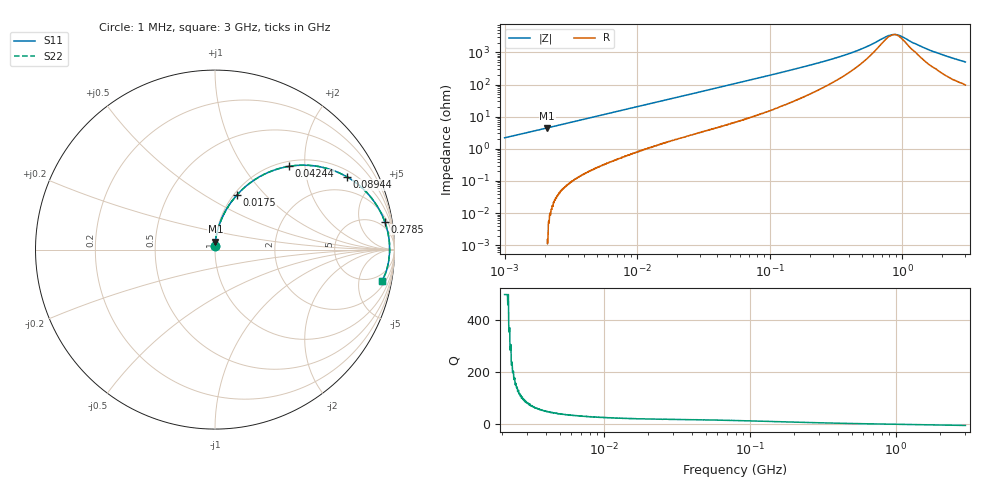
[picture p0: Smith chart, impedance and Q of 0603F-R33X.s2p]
!s-Parameter Generated by FASTRON Sdn. Bhd.
!FASTRON P/N : 0603F-R33X
!Keysight Technologies: E4991B_MY54100416_A.01.15
!Date: Thu Jun 20 13:22:18 2024
!Version  :Rev00  Thu Jun 20 13:22:18 2024
!Data & Calibration Information:
!Freq  S11  S21  S12  S22
!PortZ  Port1:50+j0  Port2:50+j0
!When reading reference impedance value at option line is always used.
! Remarks : This data is being provided solely for informational purposes.
# Hz S dB R 50
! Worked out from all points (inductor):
!   1601 points, 1 MHz to 3 GHz, reference 50 ohm
!   read as one part in series: L = 346 nH near 1.041 MHz
!   highest Q = 372 at 2.097 MHz (marker M1), where L = 340 nH
!   self-resonance near 872.6 MHz
!   S11 on the Smith chart (normalised r, x): 1 MHz: 1.00, +0.04; 17.5 MHz: 1.03, +0.70; 42.44 MHz: 1.10, +1.66; 89.44 MHz: 1.26, +3.46; 278.5 MHz: 3, +11; 3 GHz: 3, -10
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1000000  -33.10 91.5  0.01 -1.3  0.01 -1.3  -33.10 91.5
2097170  -27.00 87.4  -0.01 -2.6  -0.01 -2.6  -27.00 87.4
3804036  -22.00 84.4  -0.04 -4.6  -0.04 -4.6  -22.00 84.4
7550455  -16.30 79.3  -0.15 -8.8  -0.15 -8.8  -16.30 79.3
1.447069e7  -11.10 71.3  -0.46 -16.1  -0.46 -16.1  -11.10 71.3
1.750132e7  -9.70 68.1  -0.64 -19.1  -0.64 -19.1  -9.70 68.1
2.718395e7  -6.66 59.3  -1.30 -27.6  -1.30 -27.6  -6.66 59.3
4.243531e7  -4.12 48.3  -2.53 -38.4  -2.53 -38.4  -4.12 48.3
5.504702e7  -2.98 41.3  -3.59 -45.1  -3.59 -45.1  -2.98 41.3
8.944052e7  -1.52 28.8  -6.31 -56.9  -6.31 -56.9  -1.52 28.8
1.341416e8  -0.85 20.2  -9.21 -64.5  -9.21 -64.5  -0.85 20.2
2.083556e8  -0.49 13.0  -12.90 -69.5  -12.90 -69.5  -0.49 13.0
2.785165e8  -0.37 9.4  -15.60 -70.8  -15.60 -70.8  -0.37 9.4
4.75755e8  -0.26 4.3  -21.90 -66.0  -21.90 -66.0  -0.26 4.3
5.696638e8  -0.25 3.0  -24.70 -59.6  -24.70 -59.6  -0.25 3.0
7.925923e8  -0.24 0.6  -30.70 -21.0  -30.70 -21.0  -0.24 0.6
8.71647e8  -0.24 0.0  -31.40 -0.3  -31.40 -0.3  -0.24 0.0
9.490412e8  -0.24 -0.6  -30.80 20.1  -30.80 20.1  -0.24 -0.6
1.194682e9  -0.26 -2.2  -26.40 51.4  -26.40 51.4  -0.26 -2.2
1.662201e9  -0.28 -4.7  -21.30 65.9  -21.30 65.9  -0.28 -4.7
2.347656e9  -0.36 -7.8  -17.10 69.4  -17.10 69.4  -0.36 -7.8
3e9  -0.47 -10.6  -14.50 68.3  -14.50 68.3  -0.47 -10.6
